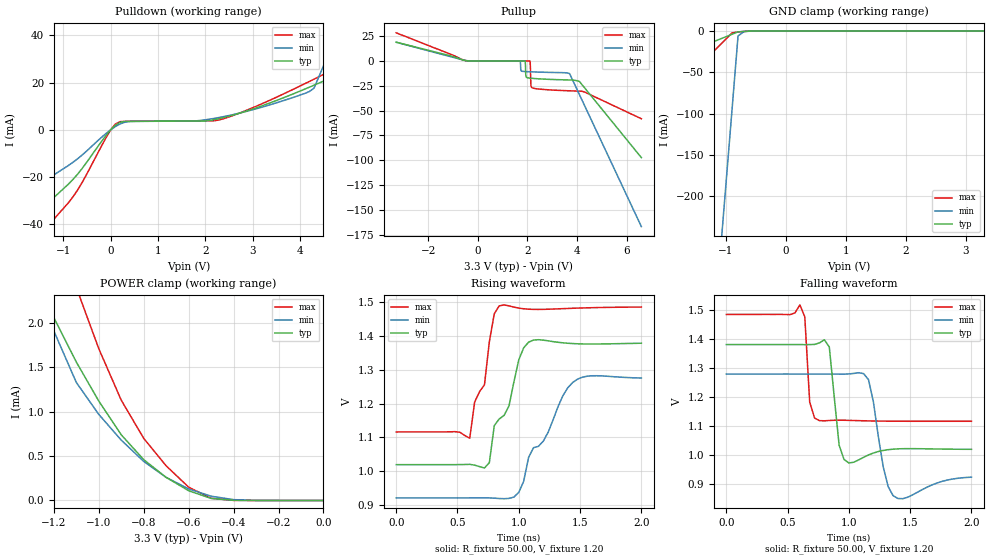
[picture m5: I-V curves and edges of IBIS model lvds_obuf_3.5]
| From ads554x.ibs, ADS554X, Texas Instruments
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|   Model lvds_obuf_3.5
[Model]   lvds_obuf_3.5
Model_type   3-state
Polarity   Non-Inverting
Enable   Active-High
Vmeas =   1.2000V
Cref =   5.0000pF
Rref = 50.0000
Vref =   1.2000V
C_comp   2.13pF   1.93pF   2.33pF
[Temperature Range]   27.00   125   -40.00
[Voltage Range]   3.30V   3.00V   3.60V
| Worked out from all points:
|   slope of the pulldown table from 0 to 0.495 V, typ, clamps not added: 136 ohm
|   GND clamp passes 1 mA (typ) near -0.79 V on its own axis
|   POWER clamp passes 1 mA (typ) near -0.97 V on its own axis
|   rising waveform, R_fixture 50.00, V_fixture 1.20: 20-80 % time 202ps typ, 285ps min, 139ps max; typ from 1.02 V to 1.38 V
|   falling waveform, R_fixture 50.00, V_fixture 1.20: 20-80 % time 51.2ps typ, 79.6ps min, 30.1ps max; typ from 1.38 V to 1.02 V
[Pulldown]
| voltage   I(typ)   I(min)   I(max)
-3.3V     -67.38mA   -46.24mA   -85.38mA
-2.1V     -45.3mA    -30.76mA   -58.26mA
-1.5V     -34.26mA   -23.02mA   -44.7mA
-800mV    -21.18mA   -13.88mA   -28.58mA
200mV     3.14mA     2.43mA     3.42mA
2.4V      5.2mA      5.59mA     4.74mA
4.3V      18.85mA    17.62mA    21.42mA
4.7V      22.5mA     36.54mA    25.45mA
4.9V      28.73mA    46mA       27.49mA
5.1V      47.65mA    55.46mA    29.72mA
5.5V      85.49mA    74.38mA    60.34mA
6.6V      189.6mA    126.4mA    178.9mA
[Pullup]
| voltage   I(typ)   I(min)   I(max)
-3.3V     18.97mA    18.87mA    28.41mA
-500mV    360uA      560uA      330uA
1.7V      27.01uA    11.29uA    46.56uA
1.74V     25.18uA    -9.712mA   44.22uA
1.9V      13.86uA    -10.6mA    34.81uA
1.94V     -15.64mA   -10.66mA   32.45uA
2.1V      -17.29mA   -10.86mA   -11.67uA
2.14V     -17.39mA   -10.91mA   -24.93mA
2.18V     -17.48mA   -10.95mA   -26.83mA
3.7V      -19.14mA   -12.67mA   -30.04mA
4.1V      -20.68mA   -33.95mA   -30.35mA
6.6V      -97.43mA   -166.9mA   -58.23mA
[GND_clamp]
| voltage   I(typ)   I(min)   I(max)
-3.3V     -73.53mA   -2.228A    -176.7mA
-1.1V     -9.73mA    -272.6mA   -16.77mA
-1V       -6.83mA    -183.7mA   -9.5mA
-900mV    -3.93mA    -94.8mA    -2.23mA
-800mV    -1.03mA    -5.92mA    -1.19mA
-700mV    -450uA     -730uA     -490uA
3.3V      44.64pA    1.08uA     37.43pA
[POWER_clamp]
| voltage   I(typ)   I(min)   I(max)
-3.3V     247.8mA    491.9mA    558.7mA
-1.3V     2.62mA     3.21mA     3.99mA
-1.2V     2.06mA     1.91mA     3.16mA
-1.1V     1.56mA     1.33mA     2.4mA
-1V       1.12mA     970uA      1.71mA
-900mV    740uA      680uA      1.13mA
-800mV    460uA      440uA      700uA
-700mV    260uA      260uA      390uA
-600mV    110uA      130uA      150uA
-500mV    23.34uA    48.47uA    24.97uA
-400mV    2uA        9.55uA     1.31uA
0V        44.64pA    500pA      43.31pA
[Ramp]
| variable   typ   min   max
dV/dt_r   1.84/71.07p   1.61/0.12n   2.05/47.79p
dV/dt_f   1.58/0.13n   1.49/0.16n   1.62/0.22n
R_load = 1.00k
[Rising Waveform]
R_fixture = 50.00
V_fixture = 1.20
V_fixture_min = 1.10
V_fixture_max = 1.30
| time   V(typ)   V(min)   V(max)
0s        1.02V      921.4mV    1.116V
600ps     1.021V     921.4mV    1.098V
640ps     1.018V     921.5mV    1.205V
720ps     1.01V      921.5mV    1.256V
760ps     1.026V     921.4mV    1.383V
840ps     1.155V     919.6mV    1.489V
1ns       1.33V      937.7mV    1.482V
1.08ns    1.382V     1.041V     1.479V
1.44ns    1.378V     1.263V     1.482V
2ns       1.379V     1.276V     1.486V
[Falling Waveform]
R_fixture = 50.00
V_fixture = 1.20
V_fixture_min = 1.10
V_fixture_max = 1.30
| time   V(typ)   V(min)   V(max)
0s        1.381V     1.279V     1.484V
600ps     1.381V     1.279V     1.517V
640ps     1.38V      1.279V     1.476V
680ps     1.381V     1.279V     1.183V
800ps     1.397V     1.279V     1.118V
920ps     1.034V     1.279V     1.12V
1ns       972.6mV    1.28V      1.119V
1.16ns    1V         1.26V      1.118V
1.36ns    1.02V      860.3mV    1.117V
2ns       1.02V      923.8mV    1.116V
